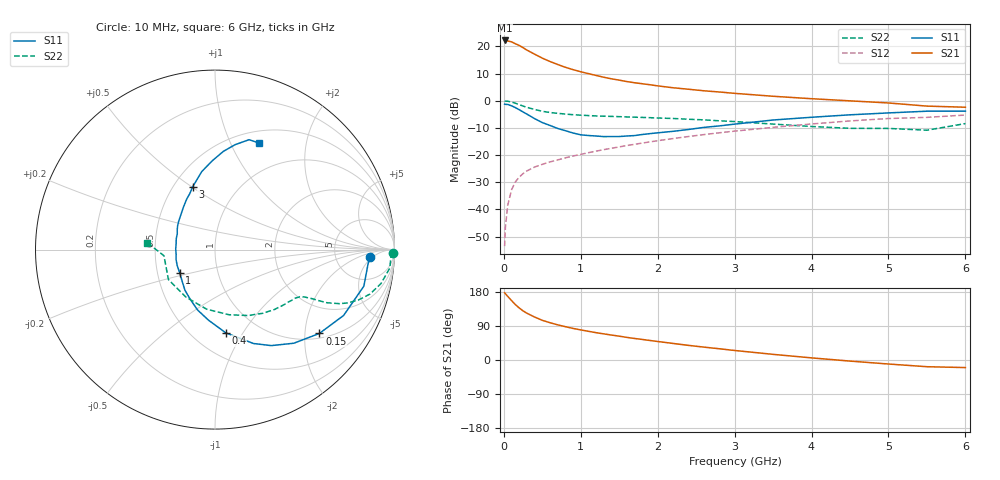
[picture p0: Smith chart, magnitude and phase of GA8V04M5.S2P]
! Infineon Technologies  Discrete & RF Semiconductors
! BF775
! Si NPN RF Bipolar Junction Transistor in SOT23
! VCE = 8 V  IC = 4.5 mA
! Common Emitter S-Parameters:  May  1996
# GHz  S  MA  R  50
!  f  S11  S21  S12  S22
! GHz  MAG  ANG  MAG  ANG  MAG  ANG  MAG  ANG
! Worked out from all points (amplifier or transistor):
!   36 points, 10 MHz to 6 GHz, reference 50 ohm
!   highest |S21| = 22.2 dB at 10 MHz (marker M1)
!   |S21| within 3 dB of that: start of sweep to 269 MHz
!   unconditionally stable (mu >= 1): 886.2 MHz to 3.041 GHz
!   at 250 MHz: K = 0.45, MSG = 23.2 dB, |S12| = -26.8 dB
!   at 1.4 GHz: K = 1.11, MAG = 10.8 dB, |S12| = -17.5 dB
!   at 6 GHz: K = 0.91, MSG = 1.4 dB, |S12| = -5.3 dB
!   S11 on the Smith chart (normalised r, x): 10 MHz: 12, -4; 150 MHz: 1.13, -2.37; 400 MHz: 0.71, -0.84; 1 GHz: 0.65, -0.18; 3 GHz: 0.62, +0.50; 6 GHz: 0.64, +1.29
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0.01  0.863 -2.7  12.85 177.4  0.0021 91.9  0.994 -1.1
0.02  0.8563 -5.5  12.58 174.9  0.0046 91.0  0.9809 -2.4
0.05  0.854 -13.8  12.6 168.0  0.0118 82.6  0.9794 -6.0
0.1  0.8051 -27.1  12.12 156.9  0.0228 76.4  0.9446 -11.5
0.15  0.7458 -38.8  11.16 146.1  0.0321 70.1  0.8985 -16.0
0.2  0.6819 -49.9  10.39 137.3  0.0392 66.3  0.8465 -19.4
0.25  0.6202 -59.6  9.452 129.6  0.0455 62.4  0.7965 -21.9
0.3  0.5655 -67.7  8.541 123.4  0.051 60.5  0.7554 -23.5
0.4  0.4678 -82.6  7.185 113.4  0.0601 57.8  0.6899 -25.4
0.5  0.3952 -95.2  6.074 104.7  0.0674 56.9  0.6384 -26.3
0.6  0.3502 -106.1  5.266 98.4  0.0746 56.8  0.6063 -26.8
0.8  0.2805 -126.8  4.121 87.9  0.0887 57.0  0.567 -27.8
1  0.2353 -146.8  3.41 79.4  0.1027 58.2  0.5412 -29.0
1.1  0.2284 -157.4  3.148 75.7  0.1104 58.4  0.5326 -30.0
1.3  0.2181 -173.3  2.7 68.9  0.1258 58.7  0.5181 -31.9
1.6  0.2241 164.4  2.249 59.6  0.1496 58.3  0.5021 -35.6
2.2  0.273 133.9  1.73 43.7  0.2009 56.1  0.4705 -45.2
3  0.3705 109.7  1.366 25.1  0.2753 50.0  0.4132 -62.8
3.5  0.4412 99.6  1.206 14.9  0.3231 45.0  0.3712 -77.9
4.5  0.5497 85.1  0.994 -2.9  0.4242 33.1  0.3101 -121.8
5.5  0.6409 72.8  0.795 -17.7  0.4934 17.6  0.2863 -173.1
6  0.6425 67.5  0.758 -20.0  0.5446 13.3  0.3793 174.2
